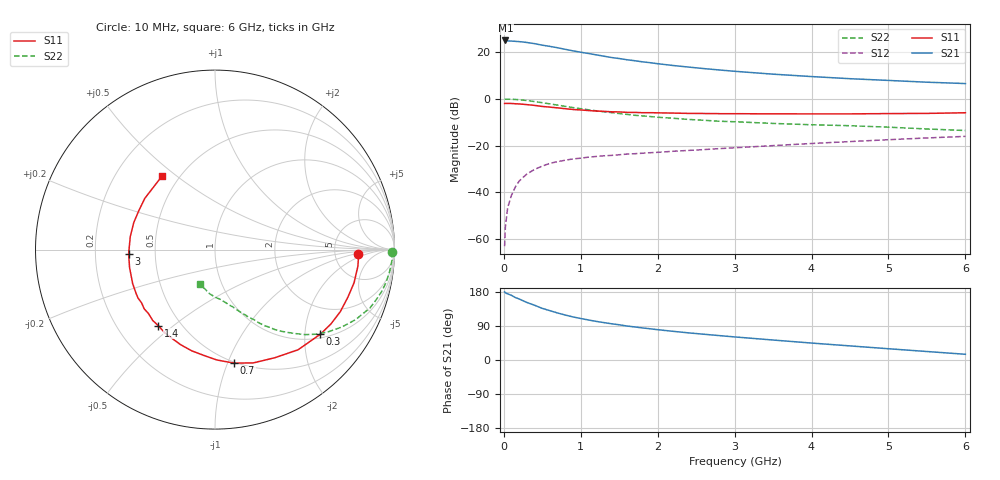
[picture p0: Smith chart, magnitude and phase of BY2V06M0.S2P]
! SIEMENS Small Signal Semiconductors
! BFY420
! Si NPN RF SIEGET Grounded Emitter Transistor in MICRO-X
! VCE = 2 V  IC = 6 mA
! Common Emitter S-Parameters:  October  1996
# GHz  S  MA  R  50
!  f  S11  S21  S12  S22
! GHz  MAG  ANG  MAG  ANG  MAG  ANG  MAG  ANG
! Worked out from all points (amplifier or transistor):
!   36 points, 10 MHz to 6 GHz, reference 50 ohm
!   highest |S21| = 25.0 dB at 20 MHz (marker M1)
!   |S21| within 3 dB of that: start of sweep to 676.5 MHz
!   unconditionally stable (mu >= 1): 2.972 GHz to end of sweep
!   at 250 MHz: K = 0.12, MSG = 29.0 dB, |S12| = -33.6 dB
!   at 1.4 GHz: K = 0.59, MSG = 21.0 dB, |S12| = -24.2 dB
!   at 6 GHz: K = 1.13, MAG = 9.1 dB, |S12| = -16.1 dB
!   S11 on the Smith chart (normalised r, x): 10 MHz: 8.80, -1.15; 300 MHz: 1.10, -2.40; 700 MHz: 0.49, -1.06; 1.4 GHz: 0.38, -0.44; 3 GHz: 0.35, -0.02; 6 GHz: 0.40, +0.44
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0.01  0.799 -1.7  17.81 179.7  0.0007 87.6  0.9882 -0.7
0.02  0.8004 -2.8  17.84 177.3  0.0018 91.9  0.9859 -1.4
0.05  0.8015 -6.6  17.44 174.5  0.0047 86.2  0.9879 -3.5
0.1  0.7965 -13.4  17.3 170.6  0.0087 84.9  0.9805 -7.2
0.15  0.7863 -19.8  17.09 164.8  0.013 79.1  0.9711 -10.7
0.2  0.7791 -26.4  16.84 161.0  0.0174 76.9  0.9584 -14.0
0.3  0.7526 -38.8  16.13 151.8  0.0246 70.5  0.9228 -20.6
0.4  0.7252 -50.3  15.24 144.4  0.0309 65.2  0.8759 -26.4
0.5  0.6883 -61.1  14.15 136.2  0.0364 60.7  0.8278 -31.4
0.6  0.6664 -71.3  13.31 130.1  0.0417 57.2  0.7806 -35.9
0.7  0.6415 -80.4  12.43 124.0  0.0453 53.8  0.735 -39.9
0.9  0.5927 -96.1  10.67 113.6  0.0518 48.1  0.6509 -46.0
1.1  0.5628 -110.1  9.387 105.6  0.0565 45.3  0.5842 -51.1
1.2  0.5488 -116.3  8.774 101.9  0.0584 44.0  0.5551 -53.3
1.4  0.5287 -126.7  7.689 95.6  0.0616 42.1  0.5082 -56.7
1.8  0.5054 -144.0  6.228 84.7  0.0685 39.7  0.4325 -62.3
2.2  0.4964 -157.5  5.19 75.7  0.0755 38.3  0.3846 -67.0
3  0.4816 -177.4  3.901 60.9  0.0897 36.8  0.3238 -74.7
3.5  0.4775 171.3  3.383 52.7  0.0998 35.3  0.2981 -79.3
4.5  0.4768 152.8  2.706 37.2  0.1218 30.9  0.2663 -89.3
5.5  0.4888 134.2  2.277 22.4  0.1456 24.6  0.2268 -104.1
6  0.5042 126.1  2.13 15.1  0.1574 21.0  0.2101 -113.5
